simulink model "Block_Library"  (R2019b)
settings: Solver=FixedStepAuto  StartTime=SimulinkInputs.t0  StopTime=SimulinkInputs.tfinal  FixedStep=1  RelTol=1e-3
undefined symbols (not defined in the file): Constants, ModelParams, SimulinkInputs

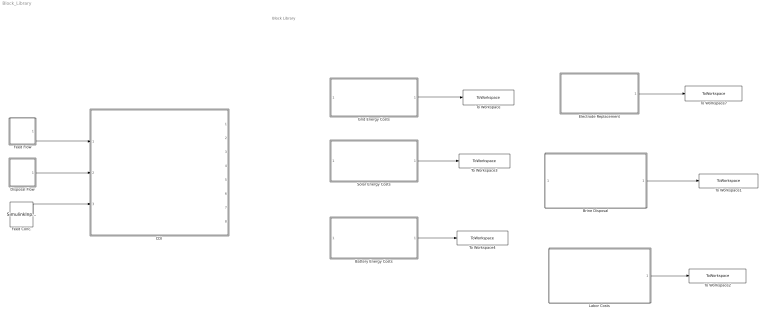
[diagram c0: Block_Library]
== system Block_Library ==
  note: Block Library
  Battery Energy Costs : Subsystem
  Brine Disposal : Subsystem
  "CDI " : Subsystem
  Disposal Flow : Subsystem
  Electrode Replacement : Subsystem
  Feed Conc. : Constant  Value=SimulinkInputs.c0
  Feed Flow : Subsystem
  Grid Energy Costs : Subsystem
  Labor Costs : Subsystem
  Solar Energy Costs : Subsystem
  To Workspace : ToWorkspace  VariableName=GridEnergyCost  SaveFormat=Timeseries  SampleTime=-1
  To Workspace1 : ToWorkspace  VariableName=DisposalCost  SaveFormat=Timeseries  SampleTime=-1
  To Workspace2 : ToWorkspace  VariableName=LaborCost  SaveFormat=Timeseries  SampleTime=-1
  To Workspace3 : ToWorkspace  VariableName=SolarEnergyCost  SaveFormat=Timeseries  SampleTime=-1
  To Workspace4 : ToWorkspace  VariableName=BatteryEnergyCost  SaveFormat=Timeseries  SampleTime=-1
  To Workspace7 : ToWorkspace  VariableName=ElectrodeCost  SaveFormat=Timeseries  SampleTime=-1
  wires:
  Solar Energy Costs/1(Out2) -> To Workspace3/1
  Battery Energy Costs/1(Out2) -> To Workspace4/1
  Electrode Replacement/1(Out1) -> To Workspace7/1
  Grid Energy Costs/1(Out1) -> To Workspace/1
  Brine Disposal/1(Out1) -> To Workspace1/1
  Labor Costs/1(Out1) -> To Workspace2/1
  Disposal Flow/1(Out1) -> "CDI "/2(In2)
  Feed Conc./1 -> "CDI "/3(In4)
  Feed Flow/1(Out1) -> "CDI "/1(In1)

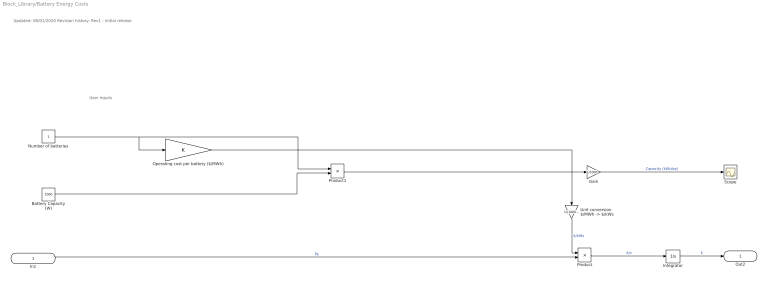
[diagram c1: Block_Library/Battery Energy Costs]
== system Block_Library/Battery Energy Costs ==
  note: User Inputs
  note: Updated: 06/01/2020 Revision history: Rev1 - initial release
  In1 : Inport
  Battery Capacity (W) : Constant  Value=1000
  Gain : Gain  Gain=1/1000
  Integrator : Integrator
  Number of batteries : Constant
  Operating cost per battery ($/MWh) : Gain
  Product : Product
  Product1 : Product
  Scope : Scope
  "Unit conversion $/MWh -> $/kWs" : Gain  Gain=1/(1000*3600)
  Out2 : Outport
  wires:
  In1/1 -> Product/2  "Pe"
  Operating cost per battery ($/MWh)/1 -> "Unit conversion $/MWh -> $/kWs"/1
  Integrator/1 -> Out2/1  "$"
  Product/1 -> Integrator/1  "$/s"
  Product1/1 -> Gain/1
  Gain/1 -> Scope/1  "Capacity (kW/day)"
  "Unit conversion $/MWh -> $/kWs"/1 -> Product/1  "$/kWs"
  Number of batteries/1 -> Operating cost per battery ($/MWh)/1, Product1/1
  Battery Capacity (W)/1 -> Product1/2

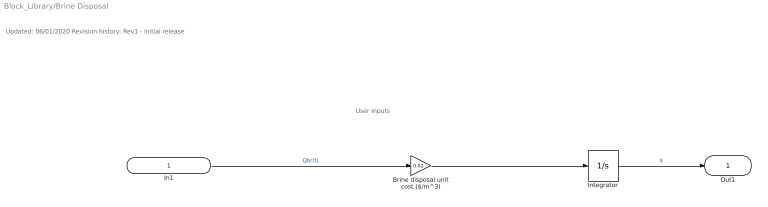
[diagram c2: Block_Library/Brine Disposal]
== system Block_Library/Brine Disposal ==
  note: User Inputs
  note: Updated: 06/01/2020 Revision history: Rev1 - initial release
  In1 : Inport
  Brine disposal unit cost ($/m^3) : Gain  Gain=0.02
  Integrator : Integrator
  Out1 : Outport  VectorParamsAs1DForOutWhenUnconnected=off
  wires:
  In1/1 -> Brine disposal unit cost ($/m^3)/1  "Qbr(t)"
  Integrator/1 -> Out1/1  "$"
  Brine disposal unit cost ($/m^3)/1 -> Integrator/1

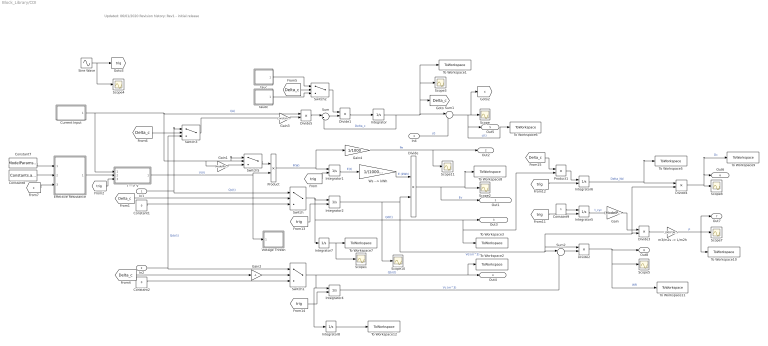
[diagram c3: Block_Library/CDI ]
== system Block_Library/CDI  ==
  note: Updated: 06/01/2020 Revision history: Rev1 - initial release
  In1 : Inport
  In2 : Inport  Port=2
  In4 : Inport  Port=3
  Constant1 : Constant  Value=0
  Constant2 : Constant  Value=0
  Constant7 : Constant  Value=ModelParams.R
  Constant8 : Constant  Value=Constants.alpha
  Constant9 : Constant
  Current Input : Subsystem
  Divide{,2,4..5} (4 alike) : Product  Inputs=*/
  Divide1 : Product  Inputs=/*
  Divide3 : Product  Inputs=/*
  Effective Resistance : MATLAB Function  TreatAsAtomicUnit=on
  Gain : Gain  Gain=(ModelParams.number_of_CDI_electrodes*ModelParams.A_CDI_electrode)
  Gain1 : Gain  Gain=ModelParams.eta_power_recovery
  Gain2 : Gain  Gain=-1
  Gain3 : Gain  Gain=Constants.F/ModelParams.Lambda_hat
  Gain4 : Gain  Gain=1/1000
  I ---> V : Subsystem
  Integrator : Integrator
  Integrator1 : Integrator  ExternalReset=rising
  Integrator2 : Integrator  ExternalReset=rising  InitialCondition=1e-12
  Integrator4 : Integrator  ExternalReset=rising
  Integrator5 : Integrator  ExternalReset=rising  InitialCondition=1
  Integrator6 : Integrator  ExternalReset=rising
  Integrator7 : Integrator
  Integrator8 : Integrator
  Product : Product
  Product1 : Product
  Scope{,1..5,7..8,10..11} (10 alike) : Scope
  Sine Wave : Sin  Frequency=(2*pi)/SimulinkInputs.Tcyc  SampleTime=0
  Sum : Sum  Inputs=|+-
  Sum1 : Sum  Inputs=|-+
  Sum2 : Sum  Inputs=|++
  Switch{,2..3,5} (4 alike) : Switch
  Switch1 : Switch  Criteria=u2 > Threshold
  To Workspace1 : ToWorkspace  VariableName=delta_c_instant  SaveFormat=Timeseries  SampleTime=-1
  To Workspace10 : ToWorkspace  VariableName=Prod  SaveFormat=Timeseries  SampleTime=-1
  To Workspace11 : ToWorkspace  VariableName=WR  SaveFormat=Timeseries  SampleTime=-1
  To Workspace12 : ToWorkspace  VariableName=Brine_Vol  SaveFormat=Timeseries  SampleTime=-1
  To Workspace2 : ToWorkspace  VariableName=Q_Brine  SaveFormat=Timeseries  SampleTime=-1
  To Workspace3 : ToWorkspace  VariableName=Q_Desal  SaveFormat=Timeseries  SampleTime=-1
  To Workspace5 : ToWorkspace  VariableName=Delta_ND  SaveFormat=Timeseries  SampleTime=-1
  To Workspace6 : ToWorkspace  VariableName=c  SaveFormat=Timeseries  SampleTime=-1
  To Workspace7 : ToWorkspace  VariableName=Desal_Vol  SaveFormat=Timeseries  SampleTime=-1
  To Workspace8 : ToWorkspace  VariableName=E_V  SaveFormat=Timeseries  SampleTime=-1
  To Workspace9 : ToWorkspace  VariableName=delta_c_average  SaveFormat=Timeseries  SampleTime=-1
  Voltage Thresh : Subsystem
  Ws --> kWh : Gain  Gain=1/(1000*3600)
  "m3/m2s -> L/m2h" : Gain  Gain=1000*3600
  tauc : Subsystem
  taudc : Subsystem
  Out1 : Outport  VectorParamsAs1DForOutWhenUnconnected=off
  Out2 : Outport  Port=2  VectorParamsAs1DForOutWhenUnconnected=off
  Out3 : Outport  Port=3  VectorParamsAs1DForOutWhenUnconnected=off
  Out4 : Outport  Port=4  VectorParamsAs1DForOutWhenUnconnected=off
  Out5 : Outport  Port=5  VectorParamsAs1DForOutWhenUnconnected=off
  Out6 : Outport  Port=6
  Out7 : Outport  Port=7
  Out8 : Outport  Port=8
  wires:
  Divide5/1 -> Sum/1
  Integrator/1 -> Sum/2, Sum1/1, To Workspace1/1, Scope3/1, [Delta_c]  "Delta_c"
  In4/1 -> Sum1/2  "c0"
  Sum1/1 -> To Workspace6/1, Out5/1, [c], Scope/1  "c(t)"
  Integrator1/1 -> Ws --> kWh/1  "E(t)"
  Divide/1 -> To Workspace8/1, Scope2/1, Out1/1  "Ev"
  [Delta_c] -> Switch/2
  Integrator2/1 -> Scope10/1, Divide4/2, Divide3/2, Divide2/1, Sum2/1, Divide/2  "Vd (m^3)"
  Switch/1 -> To Workspace3/1, Product1/2, Out3/1, Integrator7/1, Integrator2/1  "Qd(t)"
  Switch1/1 -> To Workspace2/1, Out4/1, Integrator4/1, Integrator8/1  "Qbr(t)"
  [trig] -> Integrator1/2
  Ws --> kWh/1 -> Divide/1  "E (kWh)"
  Product/1 -> Gain4/1, Integrator1/1  "P(W)"
  Gain4/1 -> Scope11/1, Out2/1  "Pe"
  Constant1/1 -> Switch/3
  Constant2/1 -> Switch1/3
  [Delta_c] -> Gain2/1
  In1/1 -> Switch/1, Switch3/1  "Qc(t)"
  Divide1/1 -> Integrator/1
  Switch2/1 -> Divide1/1
  [Delta_c] -> Switch2/2
  Sum/1 -> Divide1/2
  [Delta_c] -> Switch3/2
  Constant8/1 -> Effective Resistance/2(alpha)
  Constant7/1 -> Effective Resistance/1(R0)
  [c] -> Effective Resistance/3(c)
  Gain2/1 -> Switch1/2
  In2/1 -> Switch1/1, Switch3/3  "Qdc(t)"
  Integrator4/1 -> Sum2/2  "Vc (m^3)"
  Sum2/1 -> Divide2/2
  [trig] -> Integrator5/2
  Constant9/1 -> Integrator5/1
  Integrator5/1 -> Gain/1  "t_cyc"
  Gain/1 -> Divide3/1
  Divide3/1 -> "m3/m2s -> L/m2h"/1
  [trig] -> Integrator6/2
  Product1/1 -> Integrator6/1
  Integrator6/1 -> To Workspace5/1, Divide4/1  "Delta_Nd"
  Divide2/1 -> To Workspace11/1, Scope5/1, Out8/1  "WR"
  Divide4/1 -> To Workspace9/1, Out6/1, Scope8/1  "Dc"
  Current Input/1(Out2) -> Gain1/1, Switch5/1, Switch5/2, Divide5/1, I ---> V/1(In1)  "I(A)"
  "m3/m2s -> L/m2h"/1 -> To Workspace10/1, Out7/1, Scope7/1  "P"
  Switch3/1 -> Gain3/1
  I ---> V/1(Out1) -> Product/2, Voltage Thresh/1(In1)  "V(V)"
  Effective Resistance/1(R) -> I ---> V/2(In2)
  Switch5/1 -> Product/1
  Gain1/1 -> Switch5/3
  Integrator7/1 -> Scope1/1, To Workspace7/1
  [trig] -> Integrator2/2
  [trig] -> Integrator4/2
  [Delta_c] -> Product1/1
  Gain3/1 -> Divide5/2
  tauc/1(Out1) -> Switch2/1
  taudc/1(Out1) -> Switch2/3
  Integrator8/1 -> To Workspace12/1
  Sine Wave/1 -> Scope4/1, [trig]
  [trig] -> I ---> V/3(In3)

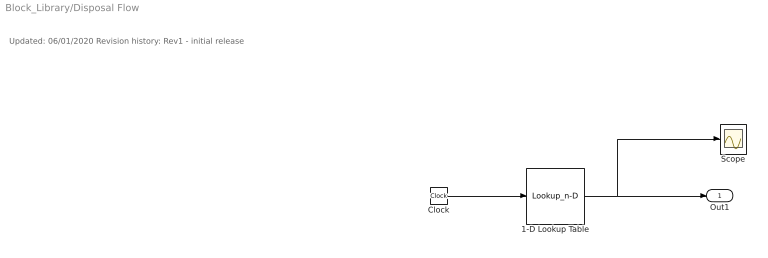
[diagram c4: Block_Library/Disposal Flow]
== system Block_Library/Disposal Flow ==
  note: Updated: 06/01/2020 Revision history: Rev1 - initial release
  1-D Lookup Table : Lookup_n-D  NumberOfTableDimensions=1  BreakpointsForDimension1=SimulinkInputs.Tvec  Table=SimulinkInputs.discharging_flowrate_timeseries  InternalRulePriority=Speed  RndMeth=Simplest
  Clock : Clock
  Scope : Scope
  Out1 : Outport
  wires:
  Clock/1 -> 1-D Lookup Table/1
  1-D Lookup Table/1 -> Out1/1, Scope/1

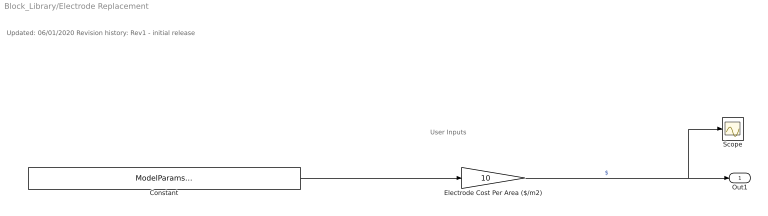
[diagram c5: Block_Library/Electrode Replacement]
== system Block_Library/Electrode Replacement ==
  note: User Inputs
  note: Updated: 06/01/2020 Revision history: Rev1 - initial release
  Constant : Constant  Value=ModelParams.number_of_CDI_electrodes*ModelParams.A_CDI_electrode
  Electrode Cost Per Area ($/m2) : Gain  Gain=10
  Scope : Scope
  Out1 : Outport
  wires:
  Electrode Cost Per Area ($/m2)/1 -> Scope/1, Out1/1  "$"
  Constant/1 -> Electrode Cost Per Area ($/m2)/1

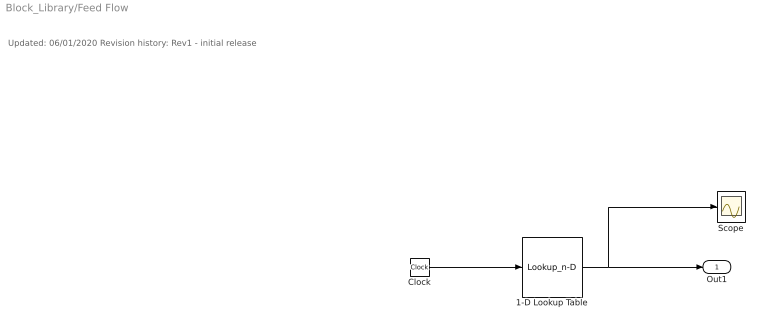
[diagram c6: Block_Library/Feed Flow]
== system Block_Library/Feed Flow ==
  note: Updated: 06/01/2020 Revision history: Rev1 - initial release
  1-D Lookup Table : Lookup_n-D  NumberOfTableDimensions=1  BreakpointsForDimension1=SimulinkInputs.Tvec  Table=SimulinkInputs.charging_flowrate_timeseries  InternalRulePriority=Speed  RndMeth=Simplest
  Clock : Clock
  Scope : Scope
  Out1 : Outport
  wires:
  Clock/1 -> 1-D Lookup Table/1
  1-D Lookup Table/1 -> Scope/1, Out1/1

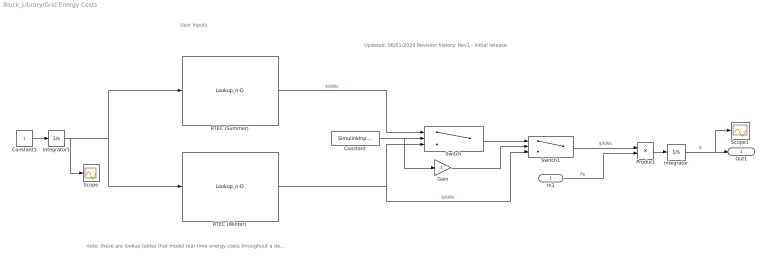
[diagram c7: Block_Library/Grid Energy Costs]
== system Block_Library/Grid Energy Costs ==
  note: note: these are lookup tables that model real-time energy costs throughout a day. Time should span from 0 to 86,400 seconds
  note: Updated: 06/01/2020 Revision history: Rev1 - initial release
  note: User Inputs
  In1 : Inport
  Constant : Constant  Value=SimulinkInputs.day
  Constant1 : Constant
  Gain : Gain  Gain=-1
  Integrator : Integrator
  Integrator1 : Integrator  InitialCondition=SimulinkInputs.t0  WrapState=on  WrappedStateUpperValue=24*3600  WrappedStateLowerValue=0
  Product : Product
  RTEC (Summer) : Lookup_n-D  NumberOfTableDimensions=1  BreakpointsForDimension1=[0;8.5;8.51;12;12.01;18;18.01;21.5;21.51;24].*3600  Table=[0.236;0.236;0.263;0.263;0.287;0.287;0.263;0.263;0.236;0.236]./(3600)  InternalRulePriority=Speed  RndMeth=Simplest
  RTEC (Winter) : Lookup_n-D  NumberOfTableDimensions=1  BreakpointsForDimension1=[0;8.5;8.51;21.5;21.51;24].*3600  Table=[0.222;0.222;0.243;0.243;0.222;0.222]./3600  InternalRulePriority=Speed  RndMeth=Simplest
  Scope : Scope
  Scope1 : Scope
  Switch : Switch  Threshold=121
  Switch1 : Switch  Threshold=-304
  Out1 : Outport  VectorParamsAs1DForOutWhenUnconnected=off
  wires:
  RTEC (Summer)/1 -> Switch/1  "$/kWs"
  RTEC (Winter)/1 -> Switch/3, Switch1/3  "$/kWs"
  Integrator1/1 -> Scope/1, RTEC (Summer)/1, RTEC (Winter)/1
  Constant/1 -> Gain/1, Switch/2
  Switch/1 -> Switch1/1
  Gain/1 -> Switch1/2
  Switch1/1 -> Product/1  "$/kWs"
  In1/1 -> Product/2  "Pe"
  Integrator/1 -> Scope1/1, Out1/1  "$"
  Product/1 -> Integrator/1
  Constant1/1 -> Integrator1/1

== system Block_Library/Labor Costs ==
  note: User Inputs
  note: Updated: 06/01/2020 Revision history: Rev1 - initial release
  Annual labor costs (% of Capital Costs per y) : Constant  Value=3
  Out1 : Outport
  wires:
  Annual labor costs (% of Capital Costs per y)/1 -> Out1/1  "%CC"

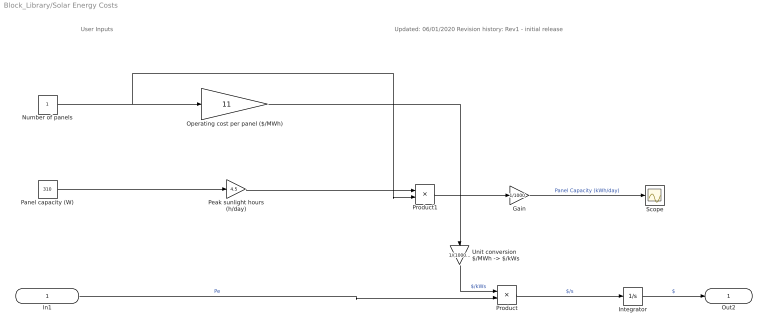
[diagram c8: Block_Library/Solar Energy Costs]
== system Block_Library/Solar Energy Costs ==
  note: User Inputs
  note: Updated: 06/01/2020 Revision history: Rev1 - initial release
  In1 : Inport
  Gain : Gain  Gain=1/1000
  Integrator : Integrator
  Number of panels : Constant
  Operating cost per panel ($/MWh) : Gain  Gain=11
  Panel capacity (W) : Constant  Value=310
  Peak sunlight hours (h/day) : Gain  Gain=4.5
  Product : Product
  Product1 : Product
  Scope : Scope
  "Unit conversion $/MWh -> $/kWs" : Gain  Gain=1/(1000*3600)
  Out2 : Outport
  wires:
  In1/1 -> Product/2  "Pe"
  Panel capacity (W)/1 -> Peak sunlight hours (h/day)/1
  Peak sunlight hours (h/day)/1 -> Product1/1
  Operating cost per panel ($/MWh)/1 -> "Unit conversion $/MWh -> $/kWs"/1
  Integrator/1 -> Out2/1  "$"
  Product/1 -> Integrator/1  "$/s"
  Product1/1 -> Gain/1
  Gain/1 -> Scope/1  "Panel Capacity (kWh/day)"
  "Unit conversion $/MWh -> $/kWs"/1 -> Product/1  "$/kWs"
  Number of panels/1 -> Operating cost per panel ($/MWh)/1, Product1/2

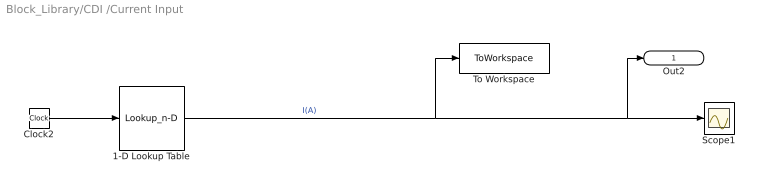
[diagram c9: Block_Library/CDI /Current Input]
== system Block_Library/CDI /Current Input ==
  1-D Lookup Table : Lookup_n-D  NumberOfTableDimensions=1  BreakpointsForDimension1=SimulinkInputs.Tvec  Table=SimulinkInputs.forcing_function_timeseries  InternalRulePriority=Speed  RndMeth=Simplest
  Clock2 : Clock
  Scope1 : Scope
  To Workspace : ToWorkspace  VariableName=Forcing_Current  SaveFormat=Timeseries  SampleTime=-1
  Out2 : Outport  VectorParamsAs1DForOutWhenUnconnected=off
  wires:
  Clock2/1 -> 1-D Lookup Table/1
  1-D Lookup Table/1 -> To Workspace/1, Out2/1, Scope1/1  "I(A)"

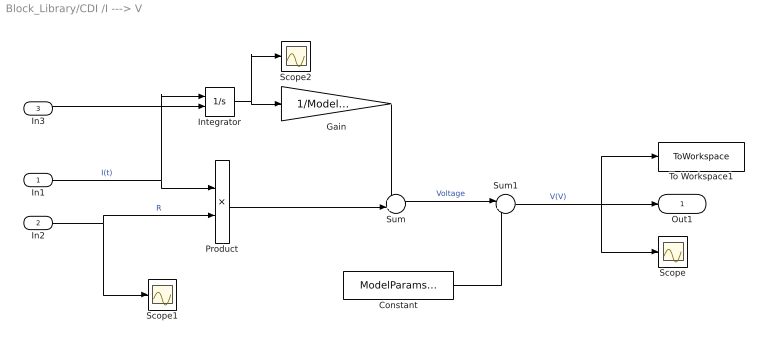
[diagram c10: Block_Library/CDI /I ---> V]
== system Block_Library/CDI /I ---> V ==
  In1 : Inport
  In2 : Inport  Port=2
  In3 : Inport  Port=3
  Constant : Constant  Value=ModelParams.V_offset
  Gain : Gain  Gain=1/ModelParams.C
  Integrator : Integrator  ExternalReset=rising
  Product : Product
  Scope : Scope
  Scope1 : Scope
  Scope2 : Scope
  Sum : Sum  Inputs=++|
  Sum1 : Sum  Inputs=|++
  To Workspace1 : ToWorkspace  VariableName=Forcing_Voltage  SaveFormat=Timeseries  SampleTime=-1
  Out1 : Outport
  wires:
  In1/1 -> Integrator/1, Product/1  "I(t)"
  In2/1 -> Scope1/1, Product/2  "R"
  Integrator/1 -> Scope2/1, Gain/1
  Product/1 -> Sum/2
  Gain/1 -> Sum/1
  Sum/1 -> Sum1/1  "Voltage"
  Constant/1 -> Sum1/2
  Sum1/1 -> Scope/1, To Workspace1/1, Out1/1  "V(V)"
  In3/1 -> Integrator/2

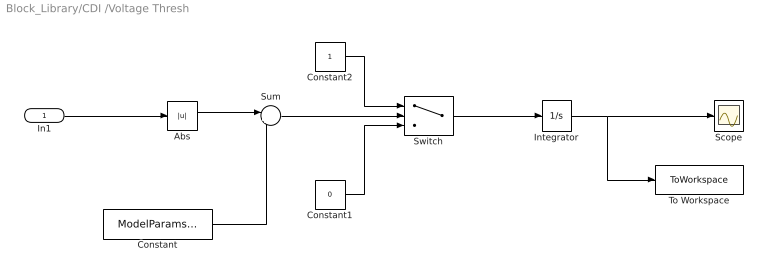
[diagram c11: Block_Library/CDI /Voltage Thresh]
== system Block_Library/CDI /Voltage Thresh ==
  In1 : Inport
  Abs : Abs
  Constant : Constant  Value=ModelParams.V_thresh
  Constant1 : Constant  Value=0
  Constant2 : Constant
  Integrator : Integrator  InitialCondition=1
  Scope : Scope
  Sum : Sum  Inputs=|+-
  Switch : Switch  Criteria=u2 > Threshold
  To Workspace : ToWorkspace  VariableName=VThreshTime  SaveFormat=Timeseries  SampleTime=-1
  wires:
  In1/1 -> Abs/1
  Abs/1 -> Sum/1
  Constant/1 -> Sum/2
  Sum/1 -> Switch/2
  Switch/1 -> Integrator/1
  Constant2/1 -> Switch/1
  Constant1/1 -> Switch/3
  Integrator/1 -> To Workspace/1, Scope/1

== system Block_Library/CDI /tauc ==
  1-D Lookup Table : Lookup_n-D  NumberOfTableDimensions=1  BreakpointsForDimension1=SimulinkInputs.Tvec  Table=SimulinkInputs.tauc_timeseries  InternalRulePriority=Speed  RndMeth=Simplest
  Clock : Clock
  Scope : Scope
  Out1 : Outport
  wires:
  Clock/1 -> 1-D Lookup Table/1
  1-D Lookup Table/1 -> Scope/1, Out1/1

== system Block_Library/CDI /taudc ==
  1-D Lookup Table : Lookup_n-D  NumberOfTableDimensions=1  BreakpointsForDimension1=SimulinkInputs.Tvec  Table=SimulinkInputs.taudc_timeseries  InternalRulePriority=Speed  RndMeth=Simplest
  Clock : Clock
  Scope : Scope
  Out1 : Outport
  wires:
  Clock/1 -> 1-D Lookup Table/1
  1-D Lookup Table/1 -> Scope/1, Out1/1

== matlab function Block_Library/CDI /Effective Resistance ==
function R = fcn(R0, alpha, c)

 R = R0*(1 + (alpha/abs(c)));
